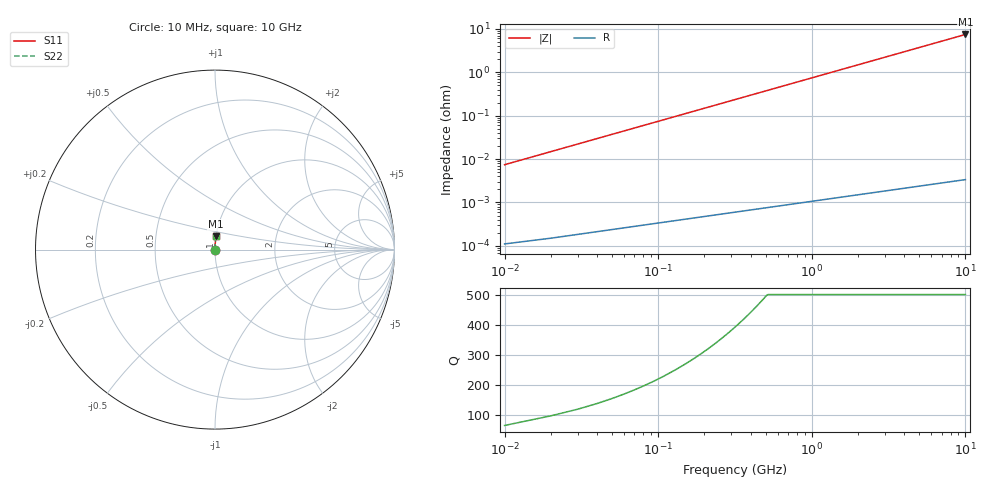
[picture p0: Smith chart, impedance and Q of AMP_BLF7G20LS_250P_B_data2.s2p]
! Created Thu Oct 28 10:33:33 2010
# ghz S ma R 50
! 2 Port Network Data from SP1.SP block
! freq  magS11  angS11  magS21  angS21  magS12  angS12  magS22  angS22
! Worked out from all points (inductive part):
!   1000 points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, 10 MHz to 10 GHz, reference 50 ohm
!   read as one part in series: L = 118 pH near 60 MHz
!   highest |Z| = 7.41 ohm at 10 GHz (marker M1)
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0.01  7.409e-05 89.1  1 -0.0  1 -0.0  7.409e-05 89.1
0.04  0.0002963 89.6  1 -0.0  1 -0.0  0.0002963 89.6
0.08  0.0005927 89.7  1 -0.0  1 -0.0  0.0005927 89.7
0.11  0.0008149 89.7  1 -0.0  1 -0.0  0.0008149 89.7
0.14  0.001037 89.7  1 -0.1  1 -0.1  0.001037 89.7
0.19  0.001408 89.7  1 -0.1  1 -0.1  0.001408 89.7
0.24  0.001778 89.7  1 -0.1  1 -0.1  0.001778 89.7
0.31  0.002297 89.7  1 -0.1  1 -0.1  0.002297 89.7
0.39  0.002889 89.7  1 -0.2  1 -0.2  0.002889 89.7
0.49  0.00363 89.7  1 -0.2  1 -0.2  0.00363 89.7
0.6  0.004445 89.6  1 -0.3  1 -0.3  0.004445 89.6
0.73  0.005408 89.6  1 -0.3  1 -0.3  0.005408 89.6
0.88  0.006519 89.5  1 -0.4  1 -0.4  0.006519 89.5
1.24  0.009186 89.4  0.9999 -0.5  0.9999 -0.5  0.009186 89.4
1.68  0.01245 89.2  0.9999 -0.7  0.9999 -0.7  0.01245 89.2
2.42  0.01793 88.9  0.9998 -1.0  0.9998 -1.0  0.01793 88.9
3.34  0.02474 88.5  0.9997 -1.4  0.9997 -1.4  0.02474 88.5
4.12  0.03051 88.2  0.9995 -1.7  0.9995 -1.7  0.03051 88.2
5.01  0.03709 87.8  0.9993 -2.1  0.9993 -2.1  0.03709 87.8
6.67  0.04935 87.1  0.9988 -2.8  0.9988 -2.8  0.04935 87.1
8.34  0.06167 86.4  0.9981 -3.5  0.9981 -3.5  0.06167 86.4
10  0.07388 85.7  0.9972 -4.2  0.9972 -4.2  0.07388 85.7
